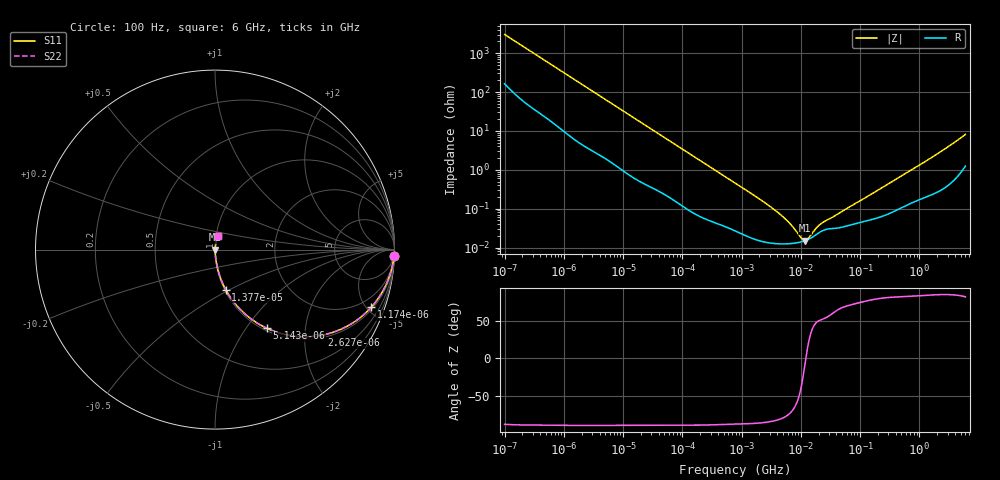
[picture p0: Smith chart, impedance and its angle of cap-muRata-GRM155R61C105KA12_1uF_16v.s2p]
!Murata Part Number: GRM155R61C105KA12
!These Parameters are Measured in Series Mode Connection
!  o--ll--o
!Port1  Port2
!  o------o
!Operation Temp=25[degC], DC Bias Voltage=0[V]
!Freq. Start=100[Hz] Stop=6[GHz], 401[Steps]
!Data Generated on Mar 6, 2017
# Hz S RI R 50
!Freq.(Hz) S11(Real) S11(Imag) S21(Real) S21(Imag) S12(Real) S12(Imag) S22(Real) S22(Imag)
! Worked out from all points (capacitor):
!   401 points, 100 Hz to 6 GHz, reference 50 ohm
!   read as one part in series: C = 526 nF near 109.4 Hz
!   lowest |Z| = 15.2 mohm at 11.89 MHz (marker M1)
!   series resonance near 12.15 MHz, so ESL is about 330 pH
!   S11 on the Smith chart (normalised r, x): 100 Hz: 4, -60; 1.174 kHz: 1.16, -5.37; 2.627 kHz: 1.07, -2.43; 5.143 kHz: 1.04, -1.26; 13.77 kHz: 1.01, -0.48; 6 GHz: 1.02, +0.16
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100  0.9971 -0.033  0.00288 0.033  0.00288 0.033  0.9971 -0.033
383.1434  0.9805 -0.1213  0.0195 0.1213  0.0195 0.1213  0.9805 -0.1213
1173.534  0.8711 -0.3206  0.1289 0.3206  0.1289 0.3206  0.8711 -0.3206
2008.354  0.7091 -0.4403  0.2909 0.4403  0.2909 0.4403  0.7091 -0.4403
2627.318  0.5931 -0.4772  0.4069 0.4772  0.4069 0.4772  0.5931 -0.4772
5142.725  0.2888 -0.4384  0.7112 0.4384  0.7112 0.4384  0.2888 -0.4384
8047.242  0.1482 -0.341  0.8518 0.341  0.8518 0.341  0.1482 -0.341
13771.83  0.0596 -0.223  0.9404 0.223  0.9404 0.223  0.0596 -0.223
40334.87  0.00958 -0.082  0.9904 0.082  0.9904 0.082  0.00958 -0.082
129199.4  0.00161 -0.0265  0.9984 0.0265  0.9984 0.0265  0.00161 -0.0265
774596.7  0.000291 -0.00459  0.9997 0.00459  0.9997 0.00459  0.000291 -0.00459
4246196  0.000126 -0.000758  0.9999 0.000758  0.9999 0.000758  0.000126 -0.000758
6644369  0.000127 -0.000386  0.9999 0.000386  0.9999 0.000386  0.000127 -0.000386
1.039699e7  0.000142 -9.37e-05  0.9999 9.37e-05  0.9999 9.37e-05  0.000142 -9.37e-05
1.189169e7  0.000151 -1.28e-05  0.9998 1.28e-05  0.9998 1.28e-05  0.000151 -1.28e-05
1.300572e7  0.00016 4.04e-05  0.9998 -4.04e-05  0.9998 -4.04e-05  0.00016 4.04e-05
1.555665e7  0.000184 0.000145  0.9998 -0.000145  0.9998 -0.000145  0.000184 0.000145
1.946e7  0.000232 0.000267  0.9998 -0.000267  0.9998 -0.000267  0.000232 0.000267
2.327686e7  0.000272 0.000345  0.9997 -0.000345  0.9997 -0.000345  0.000272 0.000345
3.124326e8  0.00077 0.00445  0.9992 -0.00445  0.9992 -0.00445  0.00077 0.00445
1.637704e9  0.00272 0.0208  0.9973 -0.0208  0.9973 -0.0208  0.00272 0.0208
6e9  0.0185 0.078  0.9815 -0.078  0.9815 -0.078  0.0185 0.078
